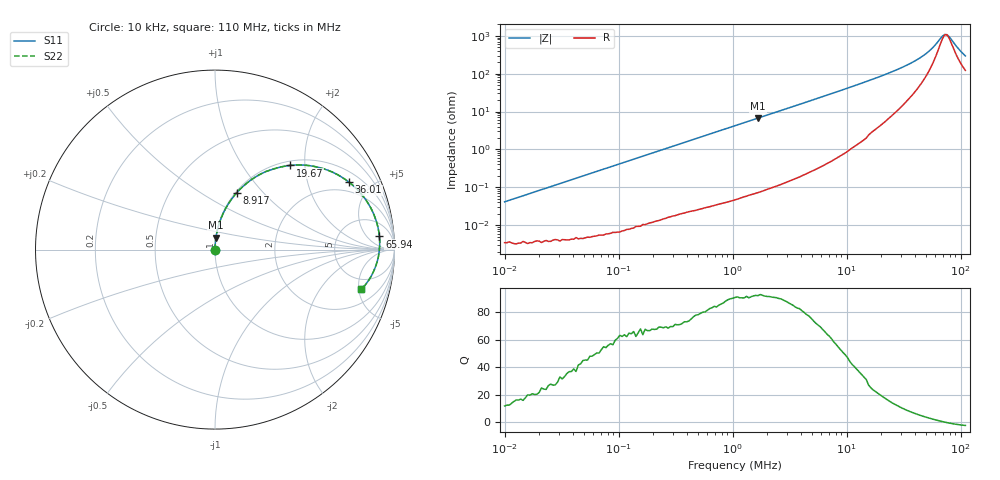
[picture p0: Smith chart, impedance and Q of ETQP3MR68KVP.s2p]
! *** S-Parameter ***
!Copyright (C)  Panasonic Industry Corporation
!Power Inductors for Automotive application
!Parts No. ETQP3MR68KVP
# HZ S RI R 50.000000
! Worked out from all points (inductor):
!   201 points, 10 kHz to 110 MHz, reference 50 ohm
!   read as one part in series: L = 655 nH near 10.48 kHz
!   highest Q = 92 at 1.67 MHz (marker M1), where L = 638 nH
!   self-resonance near 74.66 MHz
!   S11 on the Smith chart (normalised r, x): 10 kHz: 1.00, +0.00; 8.917 MHz: 1.01, +0.72; 19.67 MHz: 1.08, +1.68; 36.01 MHz: 1.47, +3.67; 65.94 MHz: 12, +12; 110 MHz: 3.44, -5.33
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10000  3.47e-05 0.000411  1 -0.000411  1 -0.000411  3.47e-05 0.000411
48644.84  4.83e-05 0.00199  1 -0.00199  1 -0.00199  4.83e-05 0.00199
225874.2  0.000217 0.00917  0.9998 -0.00917  0.9998 -0.00917  0.000217 0.00917
1048809  0.00223 0.042  0.9978 -0.042  0.9978 -0.042  0.00223 0.042
1670190  0.00518 0.0665  0.9948 -0.0665  0.9948 -0.0665  0.00518 0.0665
3058134  0.0161 0.1203  0.9839 -0.1203  0.9839 -0.1203  0.0161 0.1203
5101914  0.0426 0.1953  0.9574 -0.1953  0.9574 -0.1953  0.0426 0.1953
8916957  0.12 0.3155  0.88 -0.3155  0.88 -0.3155  0.12 0.3155
1.293816e7  0.2277 0.4059  0.7723 -0.4059  0.7723 -0.4059  0.2277 0.4059
1.966686e7  0.4196 0.4691  0.5804 -0.4691  0.5804 -0.4691  0.4196 0.4691
2.368988e7  0.5231 0.4681  0.4769 -0.4681  0.4769 -0.4681  0.5231 0.4681
2.853585e7  0.6279 0.4425  0.3721 -0.4425  0.3721 -0.4425  0.6279 0.4425
3.60102e7  0.7474 0.3752  0.2526 -0.3752  0.2526 -0.3752  0.7474 0.3752
4.337639e7  0.8251 0.2978  0.1749 -0.2978  0.1749 -0.2978  0.8251 0.2978
4.987401e7  0.8695 0.2294  0.1305 -0.2294  0.1305 -0.2294  0.8695 0.2294
5.734495e7  0.9 0.154  0.1 -0.154  0.1 -0.154  0.9 0.154
6.593501e7  0.9161 0.0735  0.0839 -0.0735  0.0839 -0.0735  0.9161 0.0735
7.236524e7  0.9173 0.0184  0.0827 -0.0184  0.0827 -0.0184  0.9173 0.0184
7.581183e7  0.9151 -0.0094  0.0849 0.0094  0.0849 0.0094  0.9151 -0.0094
7.942257e7  0.9108 -0.0374  0.0892 0.0374  0.0892 0.0374  0.9108 -0.0374
9.566912e7  0.8714 -0.1461  0.1286 0.1461  0.1286 0.1461  0.8714 -0.1461
1.1e8  0.8157 -0.2214  0.1843 0.2214  0.1843 0.2214  0.8157 -0.2214
